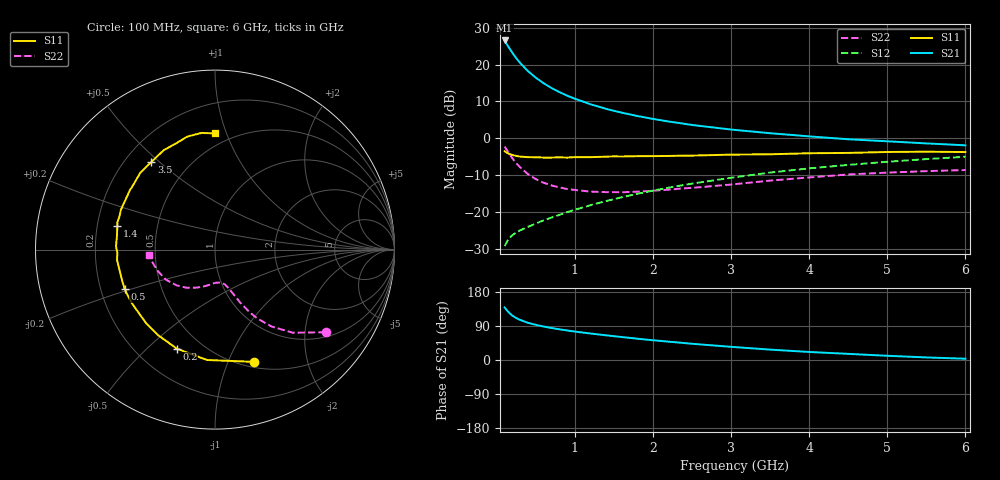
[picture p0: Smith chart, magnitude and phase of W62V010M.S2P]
! SIEMENS Small Signal Semiconductors
! BFR193W
! Si NPN RF Bipolar Junction Transistor in SOT323
! VCE = 2 V  IC = 10 mA
! Common Emitter S-Parameters:  September  1992
# GHz  S  MA  R  50
!  f  S11  S21  S12  S22
! GHz  MAG  ANG  MAG  ANG  MAG  ANG  MAG  ANG
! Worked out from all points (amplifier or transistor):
!   28 points, 100 MHz to 6 GHz, reference 50 ohm
!   highest |S21| = 26.5 dB at 100 MHz (marker M1)
!   |S21| within 3 dB of that: start of sweep to 188.6 MHz
!   unconditionally stable (mu >= 1): 970 MHz to 2.55 GHz
!   at 300 MHz: K = 0.56, MSG = 22.7 dB, |S12| = -25.0 dB
!   at 1.5 GHz: K = 1.05, MAG = 10.7 dB, |S12| = -16.6 dB
!   at 6 GHz: K = 0.91, MSG = 1.6 dB, |S12| = -5.1 dB
!   lowest NFmin = 1.30 dB at 450 MHz
!   S11 on the Smith chart (normalised r, x): 100 MHz: 0.56, -1.25; 200 MHz: 0.37, -0.62; 500 MHz: 0.30, -0.19; 1.4 GHz: 0.29, +0.11; 3.5 GHz: 0.31, +0.47; 6 GHz: 0.41, +0.92
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0.1  0.6623 -70.8  21.21 138.7  0.0341 59.8  0.7691 -36.8
0.15  0.6167 -94.2  17.33 126.0  0.0427 53.0  0.6341 -46.9
0.2  0.5913 -111.1  14.39 117.0  0.0482 49.6  0.5329 -53.6
0.25  0.5725 -123.7  12.14 110.6  0.0525 47.9  0.454 -58.2
0.3  0.5617 -133.0  10.46 105.6  0.056 47.9  0.4007 -61.0
0.4  0.5515 -147.1  8.109 98.1  0.0624 49.0  0.324 -64.7
0.5  0.5499 -156.4  6.609 92.7  0.0693 51.1  0.2775 -66.9
0.6  0.5446 -163.5  5.57 88.3  0.0765 53.0  0.2474 -69.1
0.7  0.5445 -169.0  4.792 84.4  0.0832 55.1  0.228 -70.5
0.8  0.5488 -174.1  4.232 81.0  0.0907 56.7  0.2146 -72.4
0.9  0.5443 -178.1  3.777 77.9  0.0989 58.1  0.2039 -73.6
1  0.5519 178.2  3.431 75.0  0.1065 59.3  0.198 -75.3
1.2  0.5518 171.8  2.884 69.9  0.1229 60.9  0.1877 -79.4
1.4  0.5601 166.5  2.499 65.1  0.1398 62.0  0.1849 -83.3
1.8  0.569 157.2  1.997 56.2  0.1754 62.7  0.1875 -91.7
2.2  0.5727 148.8  1.682 48.4  0.2125 62.2  0.1994 -99.4
2.5  0.579 143.0  1.509 42.8  0.2412 61.1  0.2111 -105.3
3  0.5971 134.2  1.308 34.7  0.2897 58.6  0.2344 -115.4
3.5  0.6033 126.1  1.166 27.4  0.3409 55.0  0.265 -126.6
4.5  0.6299 110.2  0.965 16.2  0.4329 46.6  0.321 -148.6
5.5  0.6544 96.5  0.848 6.8  0.5191 37.6  0.3563 -168.7
6  0.647 89.8  0.799 3.4  0.5589 32.7  0.3688 -175.7
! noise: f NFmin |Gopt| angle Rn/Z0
0.45  1.3  0.22  143  0.11
0.9  1.3  0.34  160  0.11
1.8  2.05  0.54  -153  0.14
